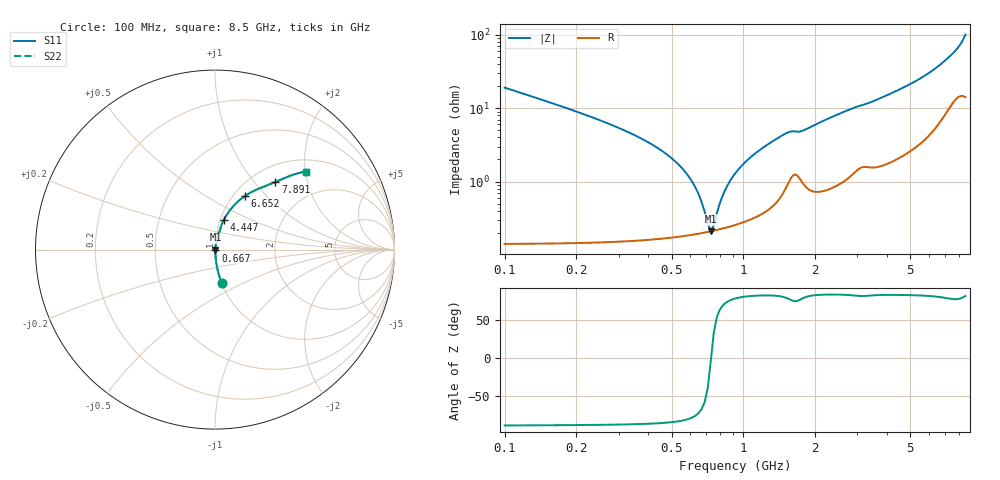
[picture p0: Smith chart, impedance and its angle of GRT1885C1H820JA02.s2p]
!Murata Part Number: GRT1885C1H820JA02
!These Parameters are Measured in Series Mode Connection
!Data Generated on Jun 19, 2026
!  o--ll--o
!Port1  Port2
!  o------o
!Operation Temp=25[degC], DC Bias Voltage=0[V]
!Freq. Start=100[MHz] Stop=9[GHz] 401[Steps]
# Hz S RI R 50
!Freq.(Hz) S11(Real) S11(Imag) S21(Real) S21(Imag) S12(Real) S12(Imag) S22(Real) S22(Imag)
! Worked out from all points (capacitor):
!   401 points, 100 MHz to 8.5 GHz, reference 50 ohm
!   read as one part in series: C = 82 pF near 142 MHz
!   lowest |Z| = 210 mohm at 730 MHz (marker M1)
!   series resonance near 732 MHz, so ESL is about 580 pH
!   S11 on the Smith chart (normalised r, x): 100 MHz: 1.00, -0.38; 667 MHz: 1.00, -0.01; 4.447 GHz: 1.04, +0.35; 6.652 GHz: 1.13, +0.77; 7.891 GHz: 1.28, +1.29; 8.5 GHz: 1.28, +2.00
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1e8  0.0363 -0.1833  0.9637 0.1833  0.9637 0.1833  0.0363 -0.1833
2.47e8  0.00629 -0.0692  0.9937 0.0692  0.9937 0.0692  0.00629 -0.0692
5.41e8  0.00204 -0.0163  0.998 0.0163  0.998 0.0163  0.00204 -0.0163
6.04e8  0.00197 -0.0103  0.998 0.0103  0.998 0.0103  0.00197 -0.0103
6.67e8  0.002 -0.00496  0.998 0.00496  0.998 0.00496  0.002 -0.00496
7.09e8  0.00206 -0.0017  0.9979 0.0017  0.9979 0.0017  0.00206 -0.0017
7.3e8  0.00209 -0.000147  0.9979 0.000147  0.9979 0.000147  0.00209 -0.000147
7.72e8  0.00219 0.00284  0.9978 -0.00284  0.9978 -0.00284  0.00219 0.00284
8.56e8  0.00244 0.00841  0.9976 -0.00841  0.9976 -0.00841  0.00244 0.00841
9.82e8  0.00298 0.016  0.997 -0.016  0.997 -0.016  0.00298 0.016
1.192e9  0.00435 0.0277  0.9956 -0.0277  0.9956 -0.0277  0.00435 0.0277
1.507e9  0.0101 0.0438  0.9899 -0.0438  0.9899 -0.0438  0.0101 0.0438
1.759e9  0.012 0.0469  0.988 -0.0469  0.988 -0.0469  0.012 0.0469
2.284e9  0.0129 0.0711  0.9871 -0.0711  0.9871 -0.0711  0.0129 0.0711
2.914e9  0.0227 0.0973  0.9773 -0.0973  0.9773 -0.0973  0.0227 0.0973
4.3e9  0.0446 0.1561  0.9554 -0.1561  0.9554 -0.1561  0.0446 0.1561
4.447e9  0.0483 0.1636  0.9517 -0.1636  0.9517 -0.1636  0.0483 0.1636
5.707e9  0.0969 0.2362  0.9031 -0.2362  0.9031 -0.2362  0.0969 0.2362
6.652e9  0.1687 0.3  0.8313 -0.3  0.8313 -0.3  0.1687 0.3
7.114e9  0.2212 0.3294  0.7788 -0.3294  0.7788 -0.3294  0.2212 0.3294
7.891e9  0.3361 0.3768  0.6639 -0.3768  0.6639 -0.3768  0.3361 0.3768
8.5e9  0.5044 0.4344  0.4956 -0.4344  0.4956 -0.4344  0.5044 0.4344
